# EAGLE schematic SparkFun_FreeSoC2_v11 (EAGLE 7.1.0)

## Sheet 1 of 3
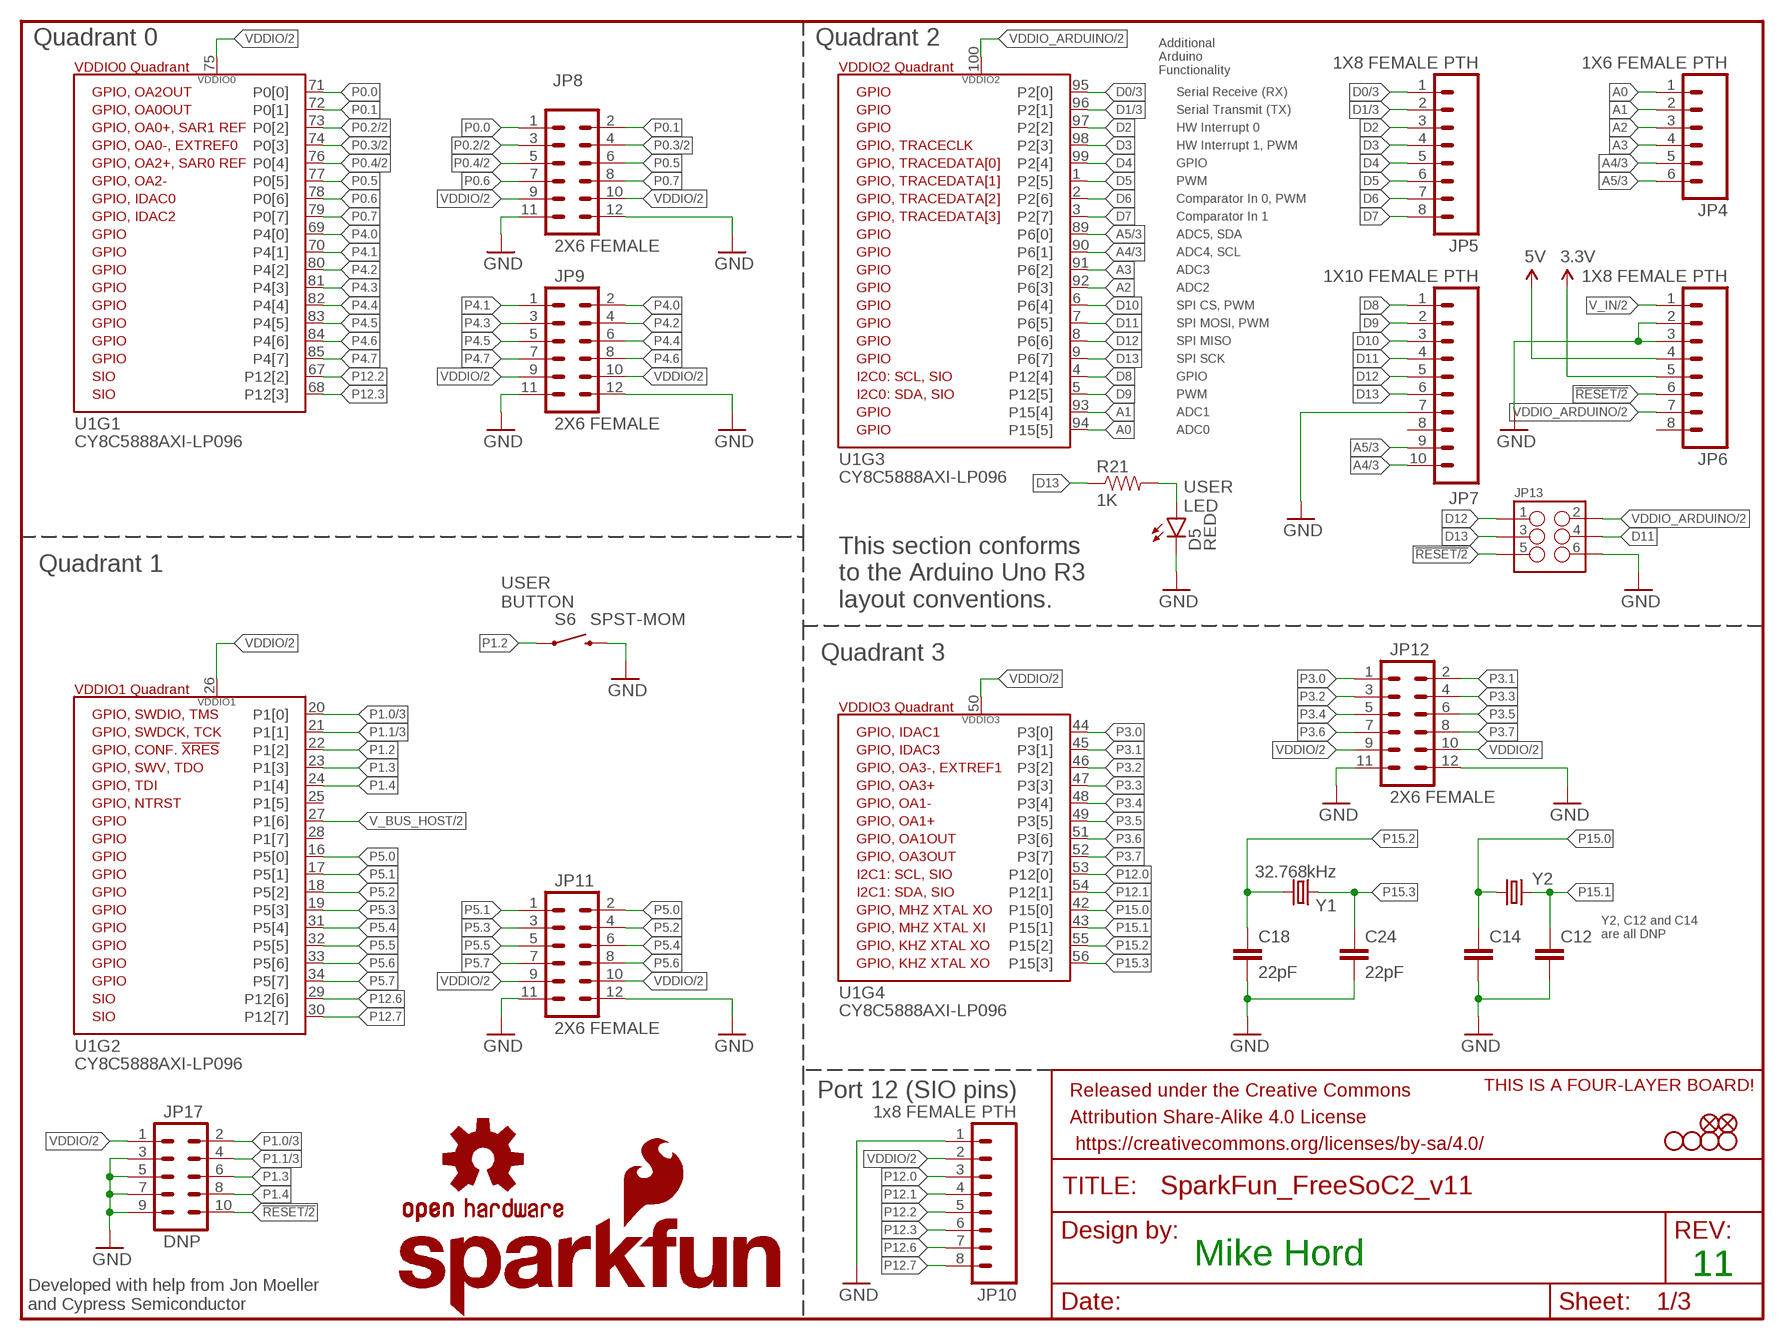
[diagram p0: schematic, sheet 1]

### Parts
C12  CAPPTH  [CAP-PTH-SMALL]
C14  CAPPTH  [CAP-PTH-SMALL]
C18  22pF  22PF-50V-5%(0603)  [0603-CAP]
C24  22pF  22PF-50V-5%(0603)  [0603-CAP]
D5  RED  LED-RED0603  [LED-0603]
FID1  FIDUCIAL1X2  [FIDUCIAL-1X2]
FID2  FIDUCIAL1X2  [FIDUCIAL-1X2]
FRAME3  FRAME-LETTERNO_PACKAGE  [DUMMY]
JP4  1X6 FEMALE PTH  M06SIP_LOCK  [1X06-SIP_LOCK]
JP5  1X8 FEMALE PTH  M08LOCK  [1X08_LOCK]
JP6  1X8 FEMALE PTH  M08LOCK  [1X08_LOCK]
JP7  1X10 FEMALE PTH  M10LOCK  [1X10_LOCK]
JP8  2X6 FEMALE  M06X2PTH_FEMALE  [2X6]
JP9  2X6 FEMALE  M06X2PTH_FEMALE  [2X6]
JP10  1x8 FEMALE PTH  M08LOCK  [1X08_LOCK]
JP11  2X6 FEMALE  M06X2PTH_FEMALE  [2X6]
JP12  2X6 FEMALE  M06X2PTH_FEMALE  [2X6]
JP13  M03X22X3_SILK_MALE_PTH  [2X3]
JP17  DNP  M05X20.05_IN_PTH_SILK  [2X5_PTH_SILK_.05]
LOGO1  SFE_LOGO_NAME_FLAME.2_INCH  [SFE_LOGO_NAME_FLAME_.2]
LOGO2  OSHW-LOGOS  [OSHW-LOGO-S]
R21  1K  1KOHM1/10W1%(0603)  [0603-RES]
S6  SPST-MOM  SWITCH-MOMENTARY-2SMD  [TACTILE-SWITCH-SMD]
STANDOFF1  STAND-OFF  [STAND-OFF]
STANDOFF2  STAND-OFF  [STAND-OFF]
STANDOFF3  STAND-OFF  [STAND-OFF]
STANDOFF4  STAND-OFF  [STAND-OFF]
U1  CY8C5888AXI-LP096  PSOC_5LP_100QFP  [TQFP-100-14X14MM]
U$1  FOUR_LAYER_WARNING  [FOUR_LAYER_WARNING]
Y1  32.768kHz  CRYSTALTC26H  [TC26H]
Y2  CRYSTALHC49US  [HC49US]

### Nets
3.3V: JP6.5 ; also sheet 2,3
5V: JP6.4 ; also sheet 2,3
!RESET: JP6.6 JP13.5 JP17.10 ; also sheet 2,3
A0: JP4.1 U1.94(P15[5])
A1: JP4.2 U1.93(P15[4])
A2: JP4.3 U1.92(P6[3])
A3: JP4.4 U1.91(P6[2])
A4: JP4.5 JP7.10 U1.90(P6[1]) ; also sheet 3
A5: JP4.6 JP7.9 U1.89(P6[0]) ; also sheet 3
D0: JP5.1 U1.95(P2[0]) ; also sheet 3
D1: JP5.2 U1.96(P2[1]) ; also sheet 3
D2: JP5.3 U1.97(P2[2])
D3: JP5.4 U1.98(P2[3])
D4: JP5.5 U1.99(P2[4])
D5: JP5.6 U1.1(P2[5])
D6: JP5.7 U1.2(P2[6])
D7: JP5.8 U1.3(P2[7])
D8: JP7.1 U1.4(P12[4])
D9: JP7.2 U1.5(P12[5])
D10: JP7.3 U1.6(P6[4])
D11: JP7.4 JP13.4 U1.7(P6[5])
D12: JP7.5 JP13.1 U1.8(P6[6])
D13: JP7.6 JP13.3 R21.1 U1.9(P6[7])
GND: C12.2 C14.2 C18.2 C24.2 D5.C JP6.2 JP6.3 JP7.7 JP8.11 JP8.12 JP9.11 JP9.12 JP10.1 JP11.11 JP11.12 JP12.11 JP12.12 JP13.6 JP17.3 JP17.5 JP17.7 JP17.9 S6.3 ; also sheet 2,3
N$26: D5.A R21.2
P0.0: JP8.1 U1.71(P0[0])
P0.1: JP8.2 U1.72(P0[1])
P0.2: JP8.3 U1.73(P0[2]) ; also sheet 2
P0.3: JP8.4 U1.74(P0[3]) ; also sheet 2
P0.4: JP8.5 U1.76(P0[4]) ; also sheet 2
P0.5: JP8.6 U1.77(P0[5])
P0.6: JP8.7 U1.78(P0[6])
P0.7: JP8.8 U1.79(P0[7])
P1.0: JP17.2 U1.20(P1[0]) ; also sheet 3
P1.1: JP17.4 U1.21(P1[1]) ; also sheet 3
P1.2: S6.1 U1.22(P1[2])
P1.3: JP17.6 U1.23(P1[3])
P1.4: JP17.8 U1.24(P1[4])
P3.0: JP12.1 U1.44(P3[0])
P3.1: JP12.2 U1.45(P3[1])
P3.2: JP12.3 U1.46(P3[2])
P3.3: JP12.4 U1.47(P3[3])
P3.4: JP12.5 U1.48(P3[4])
P3.5: JP12.6 U1.49(P3[5])
P3.6: JP12.7 U1.51(P3[6])
P3.7: JP12.8 U1.52(P3[7])
P4.0: JP9.2 U1.69(P4[0])
P4.1: JP9.1 U1.70(P4[1])
P4.2: JP9.4 U1.80(P4[2])
P4.3: JP9.3 U1.81(P4[3])
P4.4: JP9.6 U1.82(P4[4])
P4.5: JP9.5 U1.83(P4[5])
P4.6: JP9.8 U1.84(P4[6])
P4.7: JP9.7 U1.85(P4[7])
P5.0: JP11.2 U1.16(P5[0])
P5.1: JP11.1 U1.17(P5[1])
P5.2: JP11.4 U1.18(P5[2])
P5.3: JP11.3 U1.19(P5[3])
P5.4: JP11.6 U1.31(P5[4])
P5.5: JP11.5 U1.32(P5[5])
P5.6: JP11.8 U1.33(P5[6])
P5.7: JP11.7 U1.34(P5[7])
P12.0: JP10.3 U1.53(P12[0])
P12.1: JP10.4 U1.54(P12[1])
P12.2: JP10.5 U1.67(P12[2])
P12.3: JP10.6 U1.68(P12[3])
P12.6: JP10.7 U1.29(P12[6])
P12.7: JP10.8 U1.30(P12[7])
P15.0: C14.1 U1.42(P15[0]) Y2.1
P15.1: C12.1 U1.43(P15[1]) Y2.2
P15.2: C18.1 U1.55(P15[2]) Y1.2
P15.3: C24.1 U1.56(P15[3]) Y1.1
V_BUS_HOST: U1.27(P1[6]) ; also sheet 2
V_IN: JP6.1 ; also sheet 2
VDDIO: JP8.9 JP8.10 JP9.9 JP9.10 JP10.2 JP11.9 JP11.10 JP12.9 JP12.10 JP17.1 U1.26(VDDIO1) U1.50(VDDIO3) U1.75(VDDIO0) ; also sheet 2,3
VDDIO_ARDUINO [ARDUINO_VCC]: JP6.7 JP13.2 U1.100(VDDIO2) ; also sheet 2
Unconnected: JP6.8 JP7.8 U1.25(P1[5]) U1.28(P1[7])

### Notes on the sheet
- Quadrant 0 | Quadrant 2
- Additional
  Arduino
  Functionality
- Serial Receive (RX)
- Serial Transmit (TX)
- HW Interrupt 0
- HW Interrupt 1, PWM
- GPIO
- PWM
- Comparator In 0, PWM
- Comparator In 1
- ADC5, SDA
- ADC4, SCL
- ADC3
- ADC2
- SPI CS, PWM
- SPI MOSI, PWM
- SPI MISO
- SPI SCK
- GPIO
- PWM
- ADC1
- ADC0
- USER
  LED
- Quadrant 1
- USER
  BUTTON
- This section conforms
  to the Arduino Uno R3
  layout conventions.
- Quadrant 3
- Y2, C12 and C14
  are all DNP
- Port 12 (SIO pins)
- Mike Hord
- 11
- Developed with help from Jon Moeller
  and Cypress Semiconductor

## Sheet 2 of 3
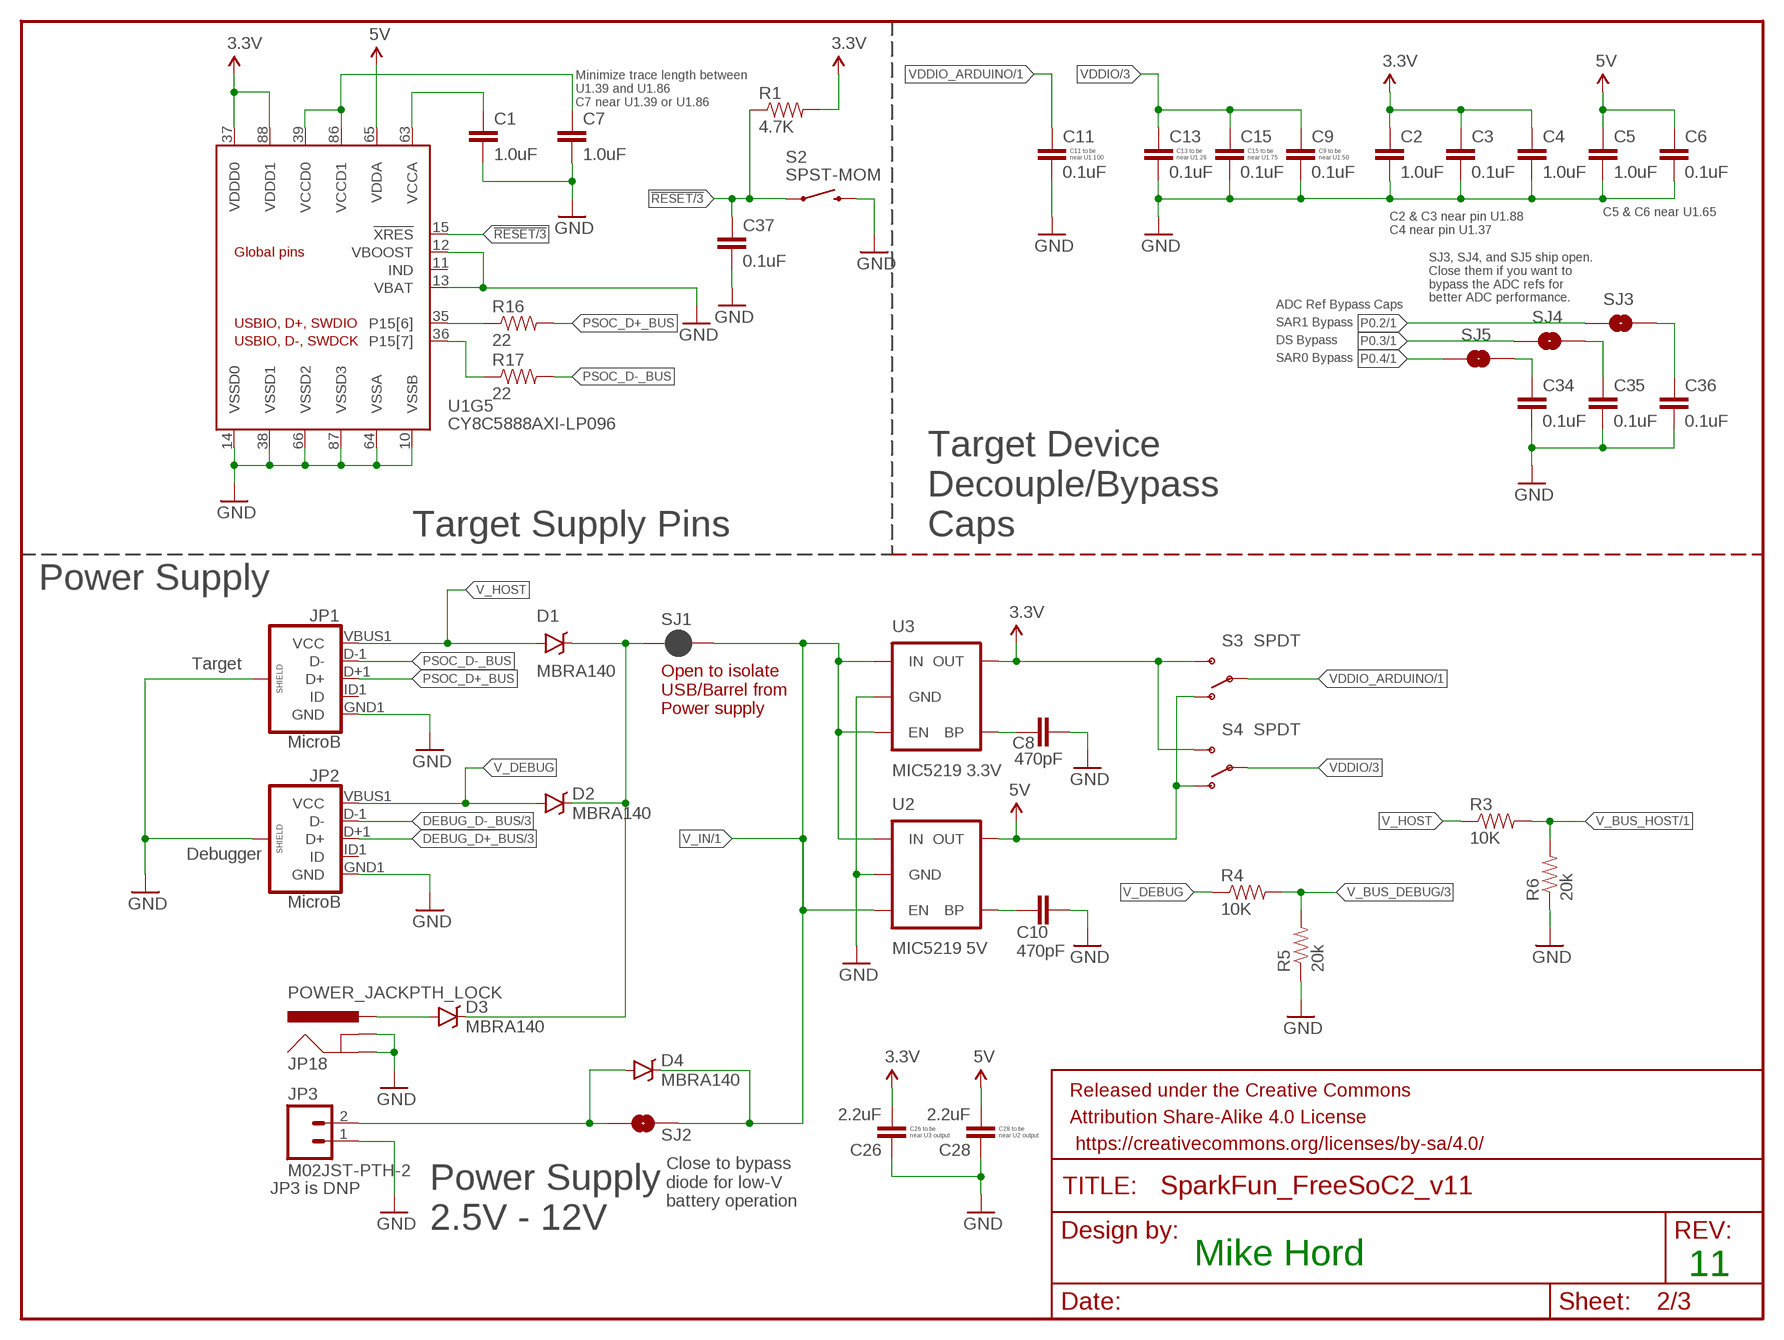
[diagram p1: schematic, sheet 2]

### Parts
C1  1.0uF  1.0UF-16V-10%(0402)  [0402-CAP]
C2  1.0uF  1.0UF-16V-10%(0402)  [0402-CAP]
C3  0.1uF  0.1UF-16V(+-10%)(0402)  [0402-CAP]
C4  1.0uF  1.0UF-16V-10%(0402)  [0402-CAP]
C5  1.0uF  1.0UF-16V-10%(0402)  [0402-CAP]
C6  0.1uF  0.1UF-16V(+-10%)(0402)  [0402-CAP]
C7  1.0uF  1.0UF-16V-10%(0402)  [0402-CAP]
C8  470pF  470PF-50V-5%(0603)SMD  [0603-CAP]
C9  0.1uF  0.1UF-16V(+-10%)(0402)  [0402-CAP]
C10  470pF  470PF-50V-5%(0603)SMD  [0603-CAP]
C11  0.1uF  0.1UF-16V(+-10%)(0402)  [0402-CAP]
C13  0.1uF  0.1UF-16V(+-10%)(0402)  [0402-CAP]
C15  0.1uF  0.1UF-16V(+-10%)(0402)  [0402-CAP]
C26  2.2uF  2.2UF-10V-20%(0603)  [0603-CAP]
C28  2.2uF  2.2UF-10V-20%(0603)  [0603-CAP]
C34  0.1uF  0.1UF-16V(+-10%)(0402)  [0402-CAP]
C35  0.1uF  0.1UF-16V(+-10%)(0402)  [0402-CAP]
C36  0.1uF  0.1UF-16V(+-10%)(0402)  [0402-CAP]
C37  0.1uF  0.1UF-16V(+-10%)(0402)  [0402-CAP]
D1  MBRA140  [SMA-DIODE]
D2  MBRA140  [SMA-DIODE]
D3  MBRA140  [SMA-DIODE]
D4  MBRA140  [SMA-DIODE]
FRAME2  FRAME-LETTERNO_PACKAGE  [DUMMY]
JP1  MicroB  USB_MICROB_PLUGCONN-11752  [USB-B-MICRO-SMD_V03]
JP2  MicroB  USB_MICROB_PLUGCONN-11752  [USB-B-MICRO-SMD_V03]
JP3  M02JST-PTH-2  [JST-2-PTH]
JP18  POWER_JACKPTH_LOCK  [POWER_JACK_PTH_LOCK]
R1  4.7K  4.7KOHM-1/10W-1%(0603)  [0603-RES]
R3  10K  10KOHM-1/10W-1%(0603)0603  [0603-RES]
R4  10K  10KOHM-1/10W-1%(0603)0603  [0603-RES]
R5  20k  20KOHM1/10W1%(0603)  [0603-RES]
R6  20k  20KOHM1/10W1%(0603)  [0603-RES]
R16  22  22OHM1/10W1%(0402)  [0402-RES]
R17  22  22OHM1/10W1%(0402)  [0402-RES]
S2  SPST-MOM  SWITCH-MOMENTARY-2SMD  [TACTILE-SWITCH-SMD]
S3  SPDT  SWITCH-SPDTPTH_LOCK  [SWITCH-SPDT_LOCK.007S]
S4  SPDT  SWITCH-SPDTPTH_LOCK  [SWITCH-SPDT_LOCK.007S]
SJ1  JUMPER-PAD-2-NC_BY_PASTE  [PAD-JUMPER-2-NC_BY_PASTE_YES_SILK]
SJ2  JUMPER-PAD-2-NOYES_SILK  [PAD-JUMPER-2-NO_YES_SILK]
SJ3  JUMPER-PAD-2-NO  [PAD-JUMPER-2-NO_NO_SILK]
SJ4  JUMPER-PAD-2-NO  [PAD-JUMPER-2-NO_NO_SILK]
SJ5  JUMPER-PAD-2-NO  [PAD-JUMPER-2-NO_NO_SILK]
U2  MIC5219 5V  V_REG_MIC52195V  [SOT23-5]
U3  MIC5219 3.3V  V_REG_MIC52193.3V  [SOT23-5]

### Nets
3.3V: C2.1 C3.1 C4.1 C26.2 R1.2 S3.3(S) S4.3(S) U1.37(VDDD0) U1.88(VDDD1) U3.5(OUT) ; also sheet 1,3
5V: C5.1 C6.1 C28.2 S3.1(O) S4.1(O) U1.65(VDDA) U2.5(OUT) ; also sheet 1,3
!RESET: C37.1 R1.1 S2.1 U1.15(!XRES) ; also sheet 1,3
DEBUG_D+_BUS: JP2.D+1(D+) ; also sheet 3
DEBUG_D-_BUS: JP2.D-1(D-) ; also sheet 3
GND: C1.2 C2.2 C3.2 C4.2 C5.2 C6.2 C7.2 C8.2 C9.2 C10.2 C11.2 C13.2 C15.2 C26.1 C28.1 C34.2 C35.2 C36.2 C37.2 JP1.GND1(GND) JP1.SHIELD1(SHIELD) JP1.SHIELD2(SHIELD) JP1.SHIELD3(SHIELD) JP2.GND1(GND) JP2.SHIELD1(SHIELD) JP2.SHIELD2(SHIELD) JP2.SHIELD3(SHIELD) JP3.1 JP18.GND JP18.GNDBREAK R5.1 R6.1 S2.3 U1.10(VSSB) U1.12(VBOOST) U1.13(VBAT) U1.14(VSSD0) U1.38(VSSD1) U1.64(VSSA) U1.66(VSSD2) U1.87(VSSD3) U2.2(GND) U3.2(GND) ; also sheet 1,3
N$1: C8.1 U3.4(BP)
N$2: C10.1 U2.4(BP)
N$3: C34.1 SJ5.2
N$4: C35.1 SJ4.2
N$5: C36.1 SJ3.2
N$13: D3.A JP18.PWR
N$16: D1.C D2.C D3.C SJ1.1
N$17: D4.A JP3.2 SJ2.1
P0.2: SJ3.1 ; also sheet 1
P0.3: SJ4.1 ; also sheet 1
P0.4: SJ5.1 ; also sheet 1
PSOC_D+_BUS: JP1.D+1(D+) R16.2
PSOC_D+_PAD: R16.1 U1.35(P15[6])
PSOC_D-_BUS: JP1.D-1(D-) R17.2
PSOC_D-_PAD: R17.1 U1.36(P15[7])
V_BUS_DEBUG: R4.2 R5.2 ; also sheet 3
V_BUS_HOST: R3.2 R6.2 ; also sheet 1
V_DEBUG: D2.A JP2.VBUS1(VCC) R4.1
V_HOST: D1.A JP1.VBUS1(VCC) R3.1
V_IN: D4.C SJ1.2 SJ2.2 U2.1(IN) U2.3(EN) U3.1(IN) U3.3(EN) ; also sheet 1
VCCA: C1.1 U1.63(VCCA)
VCCD: C7.1 U1.39(VCCD0) U1.86(VCCD1)
VDDIO: C9.1 C13.1 C15.1 S4.2(P) ; also sheet 1,3
VDDIO_ARDUINO [ARDUINO_VCC]: C11.1 S3.2(P) ; also sheet 1
Unconnected: JP1.ID1(ID) JP2.ID1(ID) U1.11(IND)

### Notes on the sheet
- Minimize trace length between
  U1.39 and U1.86
  C7 near U1.39 or U1.86
- C11 to be 
  near U1.100
- C13 to be 
  near U1.26
- C15 to be 
  near U1.75
- C9 to be 
  near U1.50
- C5 & C6 near U1.65
- C2 & C3 near pin U1.88
  C4 near pin U1.37
- SJ3, SJ4, and SJ5 ship open.
  Close them if you want to
  bypass the ADC refs for
  better ADC performance.
- ADC Ref Bypass Caps
- SAR1 Bypass
- DS Bypass
- SAR0 Bypass
- Target Supply Pins
- Target Device
  Decouple/Bypass
  Caps
- Power Supply
- Target
- Open to isolate
  USB/Barrel from
  Power supply
- Debugger
- C26 to be 
  near U3 output
- C28 to be 
  near U2 output
- JP3 is DNP
- Close to bypass
  diode for low-V
  battery operation
- Power Supply
  2.5V - 12V
- Mike Hord
- 11

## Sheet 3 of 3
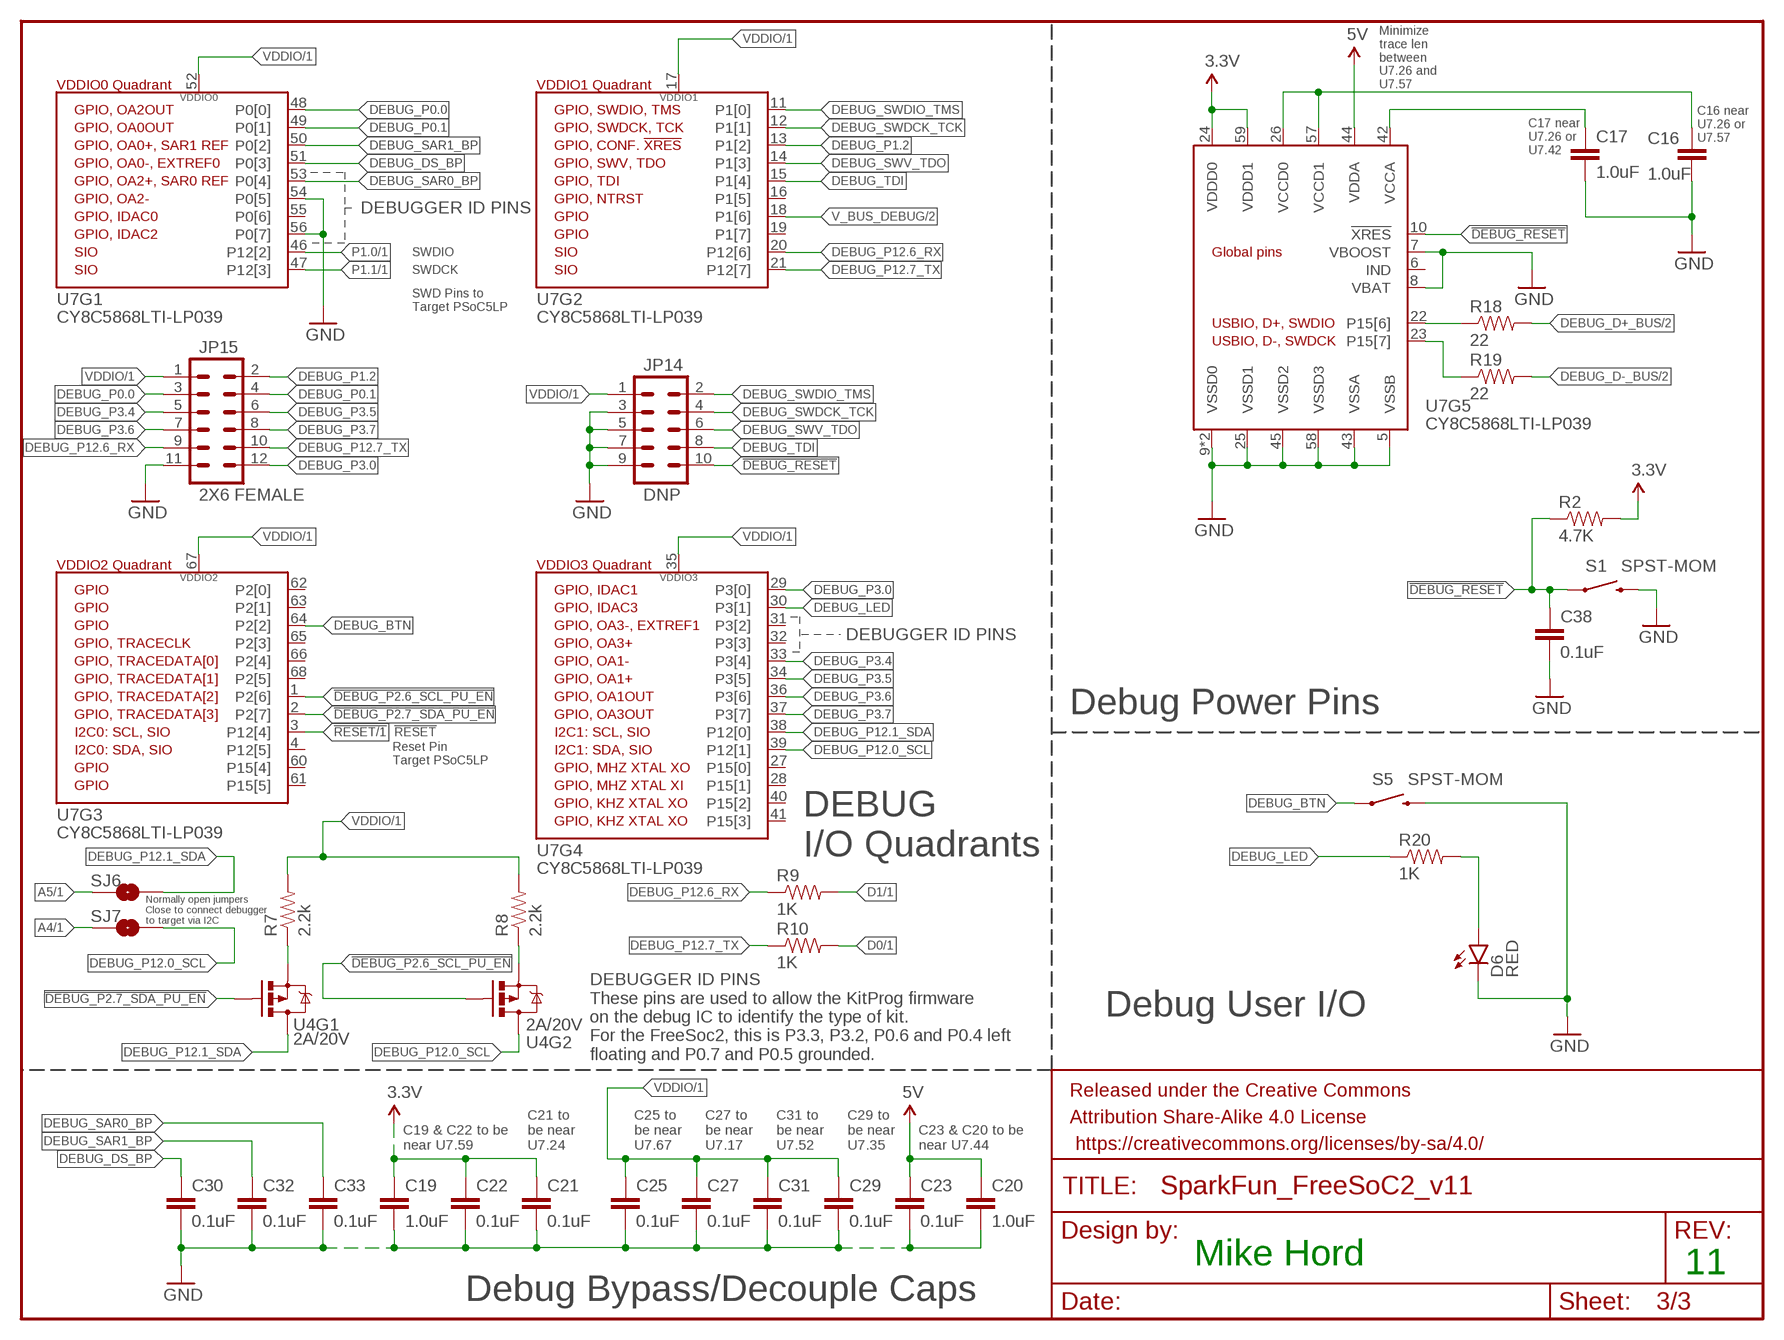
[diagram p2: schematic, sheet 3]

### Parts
C16  1.0uF  1.0UF-16V-10%(0402)  [0402-CAP]
C17  1.0uF  1.0UF-16V-10%(0402)  [0402-CAP]
C19  1.0uF  1.0UF-16V-10%(0402)  [0402-CAP]
C20  1.0uF  1.0UF-16V-10%(0402)  [0402-CAP]
C21  0.1uF  0.1UF-16V(+-10%)(0402)  [0402-CAP]
C22  0.1uF  0.1UF-16V(+-10%)(0402)  [0402-CAP]
C23  0.1uF  0.1UF-16V(+-10%)(0402)  [0402-CAP]
C25  0.1uF  0.1UF-16V(+-10%)(0402)  [0402-CAP]
C27  0.1uF  0.1UF-16V(+-10%)(0402)  [0402-CAP]
C29  0.1uF  0.1UF-16V(+-10%)(0402)  [0402-CAP]
C30  0.1uF  0.1UF-16V(+-10%)(0402)  [0402-CAP]
C31  0.1uF  0.1UF-16V(+-10%)(0402)  [0402-CAP]
C32  0.1uF  0.1UF-16V(+-10%)(0402)  [0402-CAP]
C33  0.1uF  0.1UF-16V(+-10%)(0402)  [0402-CAP]
C38  0.1uF  0.1UF-16V(+-10%)(0402)  [0402-CAP]
D6  RED  LED-RED0603  [LED-0603]
FRAME1  FRAME-LETTERNO_PACKAGE  [DUMMY]
JP14  DNP  M05X20.05_IN_PTH_SILK  [2X5_PTH_SILK_.05]
JP15  2X6 FEMALE  M06X2PTH_FEMALE  [2X6]
R2  4.7K  4.7KOHM-1/10W-1%(0603)  [0603-RES]
R7  2.2k  2.2KOHM-1/10W-1%(0603)  [0603-RES]
R8  2.2k  2.2KOHM-1/10W-1%(0603)  [0603-RES]
R9  1K  1KOHM1/10W1%(0603)  [0603-RES]
R10  1K  1KOHM1/10W1%(0603)  [0603-RES]
R18  22  22OHM1/10W1%(0402)  [0402-RES]
R19  22  22OHM1/10W1%(0402)  [0402-RES]
R20  1K  1KOHM1/10W1%(0603)  [0603-RES]
S1  SPST-MOM  SWITCH-MOMENTARY-2SMD  [TACTILE-SWITCH-SMD]
S5  SPST-MOM  SWITCH-MOMENTARY-2SMD  [TACTILE-SWITCH-SMD]
SJ6  JUMPER-PAD-2-NO  [PAD-JUMPER-2-NO_NO_SILK]
SJ7  JUMPER-PAD-2-NO  [PAD-JUMPER-2-NO_NO_SILK]
U4  2A/20V  MOSFET-PCHANNEL_DUALSOT26  [SOT26]
U7  CY8C5868LTI-LP039  PSOC_5LP_68QFN  [QFN-68]

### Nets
3.3V: C19.1 C21.1 C22.1 R2.2 U7.24(VDDD0) U7.59(VDDD1) ; also sheet 1,2
5V: C20.1 C23.1 U7.44(VDDA) ; also sheet 1,2
!DEBUG_P2.6_SCL_PU_EN: U4.G2(G) U7.1(P2[6])
!DEBUG_P2.7_SDA_PU_EN: U4.G1(G) U7.2(P2[7])
!DEBUG_RESET: C38.1 JP14.10 R2.1 S1.1 U7.10(!XRES)
!RESET: U7.3(P12[4]) ; also sheet 1,2
A4: SJ7.1 ; also sheet 1
A5: SJ6.1 ; also sheet 1
D0: R10.2 ; also sheet 1
D1: R9.2 ; also sheet 1
DEBUG_BTN: S5.1 U7.64(P2[2])
DEBUG_D+_BUS: R18.2 ; also sheet 2
DEBUG_D+_PAD: R18.1 U7.22(P15[6])
DEBUG_D-_BUS: R19.2 ; also sheet 2
DEBUG_D-_PAD: R19.1 U7.23(P15[7])
DEBUG_DS_BP: C30.1 U7.51(P0[3])
DEBUG_LED: R20.1 U7.30(P3[1])
DEBUG_P0.0: JP15.3 U7.48(P0[0])
DEBUG_P0.1: JP15.4 U7.49(P0[1])
DEBUG_P1.2: JP15.2 U7.13(P1[2])
DEBUG_P3.0: JP15.12 U7.29(P3[0])
DEBUG_P3.4: JP15.5 U7.33(P3[4])
DEBUG_P3.5: JP15.6 U7.34(P3[5])
DEBUG_P3.6: JP15.7 U7.36(P3[6])
DEBUG_P3.7: JP15.8 U7.37(P3[7])
DEBUG_P12.0_SCL: SJ7.2 U4.D2(D) U7.39(P12[1])
DEBUG_P12.1_SDA: SJ6.2 U4.D1(D) U7.38(P12[0])
DEBUG_P12.6_RX: JP15.9 R9.1 U7.20(P12[6])
DEBUG_P12.7_TX: JP15.10 R10.1 U7.21(P12[7])
DEBUG_SAR0_BP: C33.1 U7.53(P0[4])
DEBUG_SAR1_BP: C32.1 U7.50(P0[2])
DEBUG_SWDCK_TCK: JP14.4 U7.12(P1[1])
DEBUG_SWDIO_TMS: JP14.2 U7.11(P1[0])
DEBUG_SWV_TDO: JP14.6 U7.14(P1[3])
DEBUG_TDI: JP14.8 U7.15(P1[4])
GND: C16.2 C17.2 C19.2 C20.2 C21.2 C22.2 C23.2 C25.2 C27.2 C29.2 C30.2 C31.2 C32.2 C33.2 C38.2 D6.C JP14.3 JP14.5 JP14.7 JP14.9 JP15.11 S1.3 S5.3 U7.5(VSSB) U7.7(VBOOST) U7.8(VBAT) U7.9(VSSD0) U7.25(VSSD1) U7.43(VSSA) U7.45(VSSD2) U7.54(P0[5]) U7.56(P0[7]) U7.58(VSSD3) U7.69(VSSD0) ; also sheet 1,2
N$7: R8.1 U4.S2(S)
N$8: R7.1 U4.S1(S)
N$14: C16.1 U7.26(VCCD0) U7.57(VCCD1)
N$23: D6.A R20.2
N$27: C17.1 U7.42(VCCA)
P1.0: U7.46(P12[2]) ; also sheet 1
P1.1: U7.47(P12[3]) ; also sheet 1
V_BUS_DEBUG: U7.18(P1[6]) ; also sheet 2
VDDIO: C25.1 C27.1 C29.1 C31.1 JP14.1 JP15.1 R7.2 R8.2 U7.17(VDDIO1) U7.35(VDDIO3) U7.52(VDDIO0) U7.67(VDDIO2) ; also sheet 1,2
Unconnected: U7.4(P12[5]) U7.6(IND) U7.16(P1[5]) U7.19(P1[7]) U7.27(P15[0]) U7.28(P15[1]) U7.31(P3[2]) U7.32(P3[3]) U7.40(P15[2]) U7.41(P15[3]) U7.55(P0[6]) U7.60(P15[4]) U7.61(P15[5]) U7.62(P2[0]) U7.63(P2[1]) U7.65(P2[3]) U7.66(P2[4]) U7.68(P2[5])

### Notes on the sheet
- Minimize
  trace len
  between
  U7.26 and
  U7.57
- C16 near 
  U7.26 or
  U7.57
- C17 near 
  U7.26 or
  U7.42
- DEBUGGER ID PINS
- SWDIO
- SWDCK
- SWD Pins to 
  Target PSoC5LP
- DEBUGGER ID PINS
- Debug Power Pins
- !RESET
- Reset Pin
  Target PSoC5LP
- DEBUG
  I/O Quadrants
- Normally open jumpers
  Close to connect debugger
  to target via I2C
- DEBUGGER ID PINS
  These pins are used to allow the KitProg firmware
  on the debug IC to identify the type of kit. 
  For the FreeSoc2, this is P3.3, P3.2, P0.6 and P0.4 left
  floating and P0.7 and P0.5 grounded.
- Debug User I/O
- C19 & C22 to be
  near U7.59
- C21 to
  be near
  U7.24
- C25 to
  be near
  U7.67
- C27 to
  be near
  U7.17
- C31 to
  be near
  U7.52
- C29 to
  be near
  U7.35
- C23 & C20 to be
  near U7.44
- Mike Hord | 11
- Debug Bypass/Decouple Caps

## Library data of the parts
C1 C2 C4 C5 C7 C16 C17 C19 C20 = SparkFun-Capacitors:1.0UF-16V-10%(0402); PROD_ID: CAP-12417
C3 C6 C9 C11 C13 C15 C21-C23 C25 C27 C29-C38 = SparkFun-Capacitors:0.1UF-16V(+-10%)(0402); PROD_ID: CAP-12416
C8 C10 = SparkFun-Capacitors:470PF-50V-5%(0603): CAP-07884; PROD_ID: CAP-07884
C12 C14 = SparkFun-Capacitors:CAP: Capacitor
C18 C24 = SparkFun-Capacitors:22PF-50V-5%(0603): CAP-07876; PROD_ID: CAP-07876
C26 C28 = SparkFun-Capacitors:2.2UF-10V-20%(0603): CAP-07888; PROD_ID: CAP-07888
D1-D4 = SparkFun-DiscreteSemi:MBRA140: 40V, 1A Schottky rectifier; PROD_ID: DIO-08053
D5 D6 = SparkFun-LED:LED-RED: Assorted Red LEDs; PROD_ID: DIO-00819
FID1 FID2 = SparkFun-Aesthetics:FIDUCIAL: Fiducial Alignment Points
FRAME1-FRAME3 = SparkFun-Aesthetics:FRAME-LETTER: Schematic Frame; DESIGNER: Nobody; VERSION: v01
JP1 JP2 = SparkFun-Connectors:USB_MICROB_PLUG: USB Micro-B connectors Some male, some female. Watch your step!; PROD_ID: CONN-11752
JP3 = SparkFun-Connectors:M02: Standard 2-pin 0.1" header. Use with; PROD_ID: CONN-09863; SKU: PRT-09914
JP4 = SparkFun-Connectors:M06: Header 6 Standard 6-pin 0.1" header. Use with straight break away headers (SKU : PRT-00116), right angle break away headers (PRT-00553), swiss pins (PRT-00743), machine pins (PRT-00117), and female headers (PRT-00115). Molex polarized connector foot print use with SKU : PRT-08094 with associated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; PROD_ID: CONN-08437
JP5 JP6 JP10 = SparkFun-Connectors:M08: Header 8 Standard 8-pin 0.1" header. Use with straight break away headers (SKU : PRT-00116), right angle break away headers (PRT-00553), swiss pins (PRT-00743), machine pins (PRT-00117), and female headers (PRT-00115).; PROD_ID: CONN-08438
JP7 = SparkFun-Connectors:M10: Header 10 Standard 10-pin 0.1" header. Use with straight break away headers (SKU : PRT-00116), right angle break away headers (PRT-00553), swiss pins (PRT-00743), machine pins (PRT-00117), and female headers (PRT-00115).; PROD_ID: CONN-11563
JP8 JP9 JP11 JP12 JP15 = SparkFun-Connectors:M06X2; PROD_ID: CONN-12423
JP13 = SparkFun-Connectors:M03X2: 2x3 .1" header. Shrouded, with keying- CONN-10681 SMT- CONN-11415 Pogo pins- HW-11044; PROD_ID: CONN-09701
JP14 JP17 = SparkFun-Connectors:M05X2: Header 5x2 Standard 10-pin dual row 0.1" header. Commonly used with AVR-ISP. Use with Spark Fun Electronics SKU: PRT-00778
JP18 = SparkFun-Connectors:POWER_JACK: Power Jack This is the standard 5.5mm barrel jack for power. The PTH is the most common, proven, reliable, footprint. The Slot footprint only works if the mill layer is transmitted to the PCB fab house so be warned. Mating wall wart : TOL-00298 (and others); PROD_ID: CONN-08197; SF_ID: PRT-00119
LOGO1 = SparkFun-Aesthetics:SFE_LOGO_NAME_FLAME: SFE Logo, name and flame
LOGO2 = SparkFun-Aesthetics:OSHW-LOGO: Open Source Hardware Logo This logo indicates the piece of hardware it is found on incorporates a OSHW license and/or adheres to the definition of open source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
R1 R2 = SparkFun-Resistors:4.7KOHM-1/10W-1%(0603): RES-07857; PROD_ID: RES-07857
R3 R4 = SparkFun-Resistors:10KOHM-1/10W-1%(0603): RES-00824; PROD_ID: RES-00824
R5 R6 = SparkFun-Resistors:20KOHM1/10W1%(0603): RES-09383; PROD_ID: RES-09383
R7 R8 = SparkFun-Resistors:2.2KOHM-1/10W-1%(0603): RES-08272; PROD_ID: RES-08272
R9 R10 R20 R21 = SparkFun-Resistors:1KOHM1/10W1%(0603): RES-07856; PROD_ID: RES-07856
R16-R19 = SparkFun-Resistors:22OHM1/10W1%(0402); PROD_ID: RES-12427
S1 S2 S5 S6 = SparkFun-Electromechanical:SWITCH-MOMENTARY-2: Various NO switches- pushbuttons, reed, etc; PROD_ID: SWCH-08247
S3 S4 = SparkFun-Electromechanical:SWITCH-SPDT: SPDT Switch Simple slide switch, Spark Fun Electronics SKU : COM-00102 DPDT SMT slide switch, AYZ0202, SWCH-08179; PROD_ID: SWCH-08261
SJ1 = SparkFun-Passives:JUMPER-PAD-2-NC_BY_PASTE
SJ2-SJ7 = SparkFun-Passives:JUMPER-PAD-2-NO
STANDOFF1-STANDOFF4 = SparkFun-Electromechanical:STAND-OFF: #4 Stand Off
U1 = SparkFun-DigitalIC:PSOC_5LP_100QFP: Cypress PSOC 5LP, 100-pin package We use the CY8C5868AXI-LP035, which has the "full" feature set: - 256k flash - 64k SRAM - 2k EEPROM - CAN - Full-speed USB - 67MHz operation; PROD_ID: IC-12190; VALUE: CY8C5868AXI-LP035
U2 = SparkFun-PowerIC:V_REG_MIC5219: V_REG MIC5219 Standard 3.3V and 5V 500mA LDO voltage regulator in SOT-23 layout. Micrel part MIC5219. BP (by-pass) pin is used to lower output noise with 470pF cap, may be left open.; PROD_ID: VREG-10107
U3 = SparkFun-PowerIC:V_REG_MIC5219: V_REG MIC5219 Standard 3.3V and 5V 500mA LDO voltage regulator in SOT-23 layout. Micrel part MIC5219. BP (by-pass) pin is used to lower output noise with 470pF cap, may be left open.; PROD_ID: VREG-09872
U4 = SparkFun-DiscreteSemi:MOSFET-PCHANNEL_DUAL; PROD_ID: TRAN-12444
U7 = SparkFun-DigitalIC:PSOC_5LP_68QFN: PSoC5LP 68-QFN package; PROD_ID: IC-12391
U$1 = SparkFun-Aesthetics:FOUR_LAYER_WARNING: Warning text which will appear on both the schematic
Y1 = SparkFun-FreqCtrl:CRYSTAL: Various standard crystals. Proven footprints.; PROD_ID: XTAL-10112
Y2 = SparkFun-FreqCtrl:CRYSTAL: Various standard crystals. Proven footprints.

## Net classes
0 signal: width 0.203 mm, drill 0.254 mm, clearance 0.152 mm
1 AVCC: width 0.508 mm, drill 0.508 mm, clearance 0.152 mm
2 ARDUINO_VCC: width 0.508 mm, drill 0.381 mm

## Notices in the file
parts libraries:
SparkFun-Aesthetics: Licensing: Creative Commons ShareAlike 4.0 International - https://creativecommons.org/licenses/by-sa/4.0
SparkFun-Aesthetics: Released under the Creative Commons Attribution Share-Alike 4.0 License
SparkFun-Aesthetics: https://creativecommons.org/licenses/by-sa/4.0
